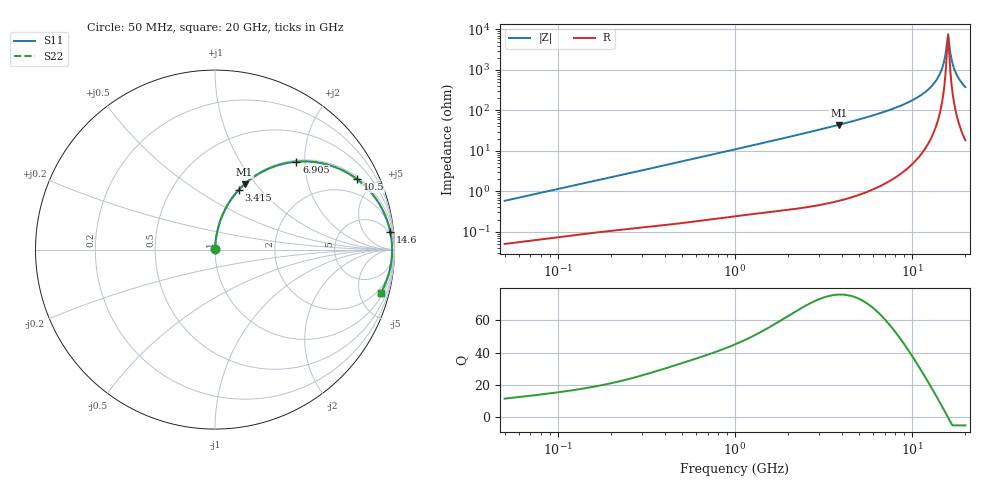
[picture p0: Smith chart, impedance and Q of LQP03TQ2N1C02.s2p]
!Murata Part Number: LQP03TQ2N1C02
!These Parameters are Measured in Series Mode Connection
!  o--[Z]--o
!Port1  Port2
!  o-------o
!Freq. Start=50[MHz] Stop=20[GHz], 401[Steps]
# Hz S RI R 50
!Freq.(Hz) S11(Real) S11(Imag) S21(Real) S21(Imag) S12(Real) S12(Imag) S22(Real) S22(Imag)
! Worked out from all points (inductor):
!   401 points, 50 MHz to 20 GHz, reference 50 ohm
!   read as one part in series: L = 1.83 nH near 51.52 MHz
!   highest Q = 75.8 at 3.85 GHz (marker M1), where L = 1.81 nH
!   self-resonance near 15.74 GHz
!   S11 on the Smith chart (normalised r, x): 50 MHz: 1.00, +0.01; 3.415 GHz: 1.01, +0.77; 6.905 GHz: 1.03, +1.82; 10.5 GHz: 1.12, +3.97; 14.6 GHz: 3, +19; 20 GHz: 1.36, -7.50
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5e7  0.000533 0.00578  0.9995 -0.00578  0.9995 -0.00578  0.000533 0.00578
1.364002e8  0.0011 0.0153  0.9989 -0.0153  0.9989 -0.0153  0.0011 0.0153
3.721004e8  0.00306 0.0406  0.9969 -0.0406  0.9969 -0.0406  0.00306 0.0406
1e9  0.014 0.1069  0.986 -0.1069  0.986 -0.1069  0.014 0.1069
2.728004e9  0.0867 0.2744  0.9133 -0.2744  0.9133 -0.2744  0.0867 0.2744
3.415248e9  0.1318 0.3317  0.8682 -0.3317  0.8682 -0.3317  0.1318 0.3317
3.850025e9  0.1645 0.3642  0.8355 -0.3642  0.8355 -0.3642  0.1645 0.3642
6.905011e9  0.454 0.4898  0.546 -0.4898  0.546 -0.4898  0.454 0.4898
7.442007e9  0.5094 0.4913  0.4906 -0.4913  0.4906 -0.4913  0.5094 0.4913
1.050288e10  0.7907 0.3925  0.2093 -0.3925  0.2093 -0.3925  0.7907 0.3925
1.295331e10  0.9316 0.2259  0.0684 -0.2259  0.0684 -0.2259  0.9316 0.2259
1.396067e10  0.9635 0.1493  0.0365 -0.1493  0.0365 -0.1493  0.9635 0.1493
1.460232e10  0.9764 0.1003  0.0236 -0.1003  0.0236 -0.1003  0.9764 0.1003
1.504638e10  0.9822 0.0669  0.0178 -0.0669  0.0178 -0.0669  0.9822 0.0669
1.550395e10  0.9857 0.033  0.0143 -0.033  0.0143 -0.033  0.9857 0.033
1.573793e10  0.9866 0.016  0.0134 -0.016  0.0134 -0.016  0.9866 0.016
1.597544e10  0.9869 -0.00104  0.0131 0.00104  0.0131 0.00104  0.9869 -0.00104
1.621653e10  0.9866 -0.0181  0.0134 0.0181  0.0134 0.0181  0.9866 -0.0181
1.696185e10  0.9822 -0.069  0.0178 0.069  0.0178 0.069  0.9822 -0.069
1.774144e10  0.9726 -0.1189  0.0274 0.1189  0.0274 0.1189  0.9726 -0.1189
1.88369e10  0.9521 -0.1829  0.0479 0.1829  0.0479 0.1829  0.9521 -0.1829
2e10  0.9236 -0.2426  0.0764 0.2426  0.0764 0.2426  0.9236 -0.2426
